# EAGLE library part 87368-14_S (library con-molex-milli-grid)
RECEPTACAL
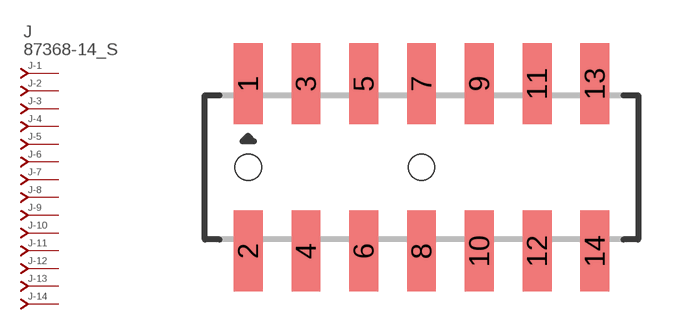
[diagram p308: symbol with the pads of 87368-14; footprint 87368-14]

Designator prefix J; gates -1=J-NV -2=J-N -3=J-N -4=J-N -5=J-N -6=J-N -7=J-N -8=J-N -9=J-N -10=J-N -11=J-N -12=J-N -13=J-N -14=J-N

## 87368-14_S  [87368-14]
1  -1:J  pas
2  -2:J  pas
3  -3:J  pas
4  -4:J  pas
5  -5:J  pas
6  -6:J  pas
7  -7:J  pas
8  -8:J  pas
9  -9:J  pas
10  -10:J  pas
11  -11:J  pas
12  -12:J  pas
13  -13:J  pas
14  -14:J  pas

## Footprint 87368-14 (pad centres in mm)
RECEPTACAL SMD Dual Row, Side Entry
smd 1 x 2.8: 1 -6,2.9; 2 -6,-2.9; 3 -4,2.9; 4 -4,-2.9; 5 -2,2.9; 6 -2,-2.9; 7 0,2.9; 8 0,-2.9; 9 2,2.9; 10 2,-2.9; 11 4,2.9; 12 4,-2.9; 13 6,2.9; 14 6,-2.9
hole 0.914 at -6,0
hole 0.914 at 0,0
